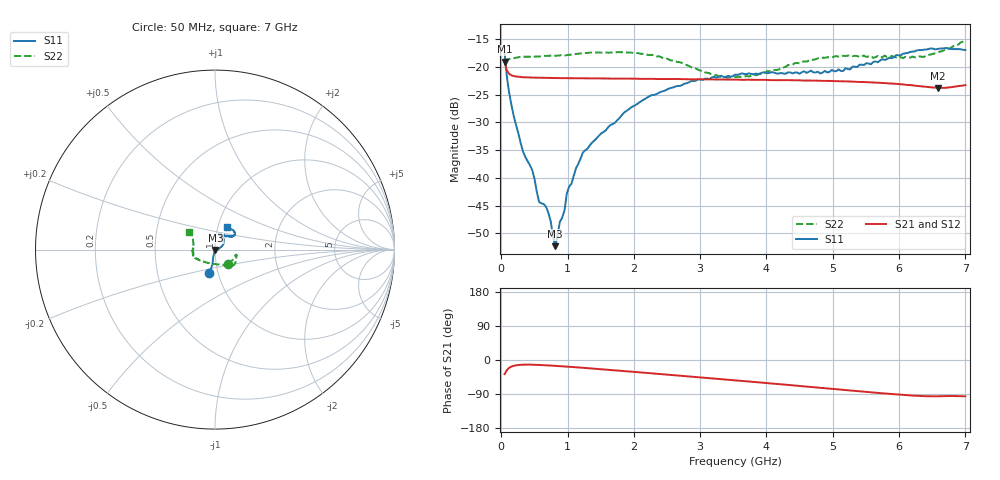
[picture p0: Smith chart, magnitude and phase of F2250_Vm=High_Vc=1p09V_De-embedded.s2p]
! Integrated Device Technology
! Corporate Headquarters
! 6024 Silver Creek Valley Road
! San Jose, CA 95138  USA
! Phone:  1-408-284-8200
! Toll Free:  1-800-223-1366
! Webpage:  http://www.idt.com/
! Timing and RF Division
! 515 Groton Road, Suite 102
! Westford, MA 01886-6024
! Device:  F2250
! Description: Voltage Variable RF Attenuator
! Frequency:  50.0 -  6000.00 MHz
! Package:  3x3 mm Thin QFN Plastic Package: 16 pin
! Ports:  2 RF, 3 DC
!  Pin  1  = GND
!  Pin  2  = NC
!  Pin  3  = RF1  = Port 1
!  Pin  4  = NC
!  Pin  5  = GND
!  Pin  6  = GND
!  Pin  7  = GND
!  Pin  8  = GND
!  Pin  9  = NC
!  Pin 10  = RF2  = Port 2
!  Pin 11  = NC
!  Pin 12  = GND
!  Pin 13  = GND
!  Pin 14  = VCNTRL
!  Pin 15  = VDD
!  Pin 16  = VMODE
! Vcntrl:  1.090 Volts
! Vmode:  +3.300 Volts
! Vdd:  +3.30  Volts
! Current:  1.330 mA
! Data:  The device was measured on a the F2250 evaluation board which has
!  individual transmission lines to the RF pins.  Data was collected
!  using a calibrated network analyzer.  The evaluation board was
!  de-embedded using a TRL calibration technique.
!  The reference plane is the edge of the package pin.
! Misc:  SN 10
!  Action Tracker AT0258
! Date Measured:  2014-11-26
! Date:  2015-10-15  MJV
! Note:
!  Integrated Device Technology supplies this data as a sample of measured
!  data at the package pin for this product.  Your particular data for this
!  product may vary.
!  Data was taken at 25 degrees C.
!  Integrated Device Technology reserves the right to change this data at anytime.
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# GHz S dB R 50
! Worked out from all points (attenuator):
!   201 points, 50 MHz to 7 GHz, reference 50 ohm
!   highest |S21| = -19.02 dB at 50 MHz (marker M1); lowest = -23.8 dB at 6.583 GHz (marker M2)
!   lowest |S11| = -52.3 dB at 814.5 MHz (marker M3), VSWR 1.00, Z = 50.2 - j0.147 ohm
!   |S11| at or under -10 dB: start of sweep to end of sweep
!   |S22| runs from -21.9 to -15.2 dB; largest |S21 - S12| = 0.00028
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0.05  -17.44 -103.4  -19.02 -37.3  -19.02 -37.3  -19.14 -48.2
0.08475  -21.81 -99.6  -20.68 -26.3  -20.67 -26.3  -18.63 -25.3
0.1195  -24.70 -101.4  -21.23 -20.5  -21.23 -20.5  -18.56 -18.0
0.29325  -33.75 -100.0  -21.80 -12.7  -21.82 -12.7  -18.12 -13.7
0.467  -38.59 -106.3  -21.92 -12.4  -21.90 -12.4  -18.18 -14.6
0.57125  -44.35 -95.6  -21.93 -13.0  -21.95 -13.1  -18.10 -17.0
0.64075  -44.72 -91.2  -21.94 -13.6  -21.94 -13.6  -17.98 -18.1
0.71025  -46.29 -79.8  -21.97 -14.3  -21.96 -14.3  -17.96 -19.9
0.8145  -52.31 -37.2  -21.99 -15.4  -21.98 -15.4  -17.98 -22.4
0.884  -47.88 -22.0  -22.01 -16.2  -21.98 -16.2  -17.89 -24.5
0.9535  -45.84 -30.4  -22.00 -17.0  -22.00 -17.0  -17.93 -25.6
0.98825  -42.84 -22.0  -22.00 -17.4  -22.00 -17.5  -17.86 -26.2
1.2315  -35.42 4.9  -22.02 -20.6  -22.03 -20.6  -17.47 -30.7
1.857  -28.16 23.9  -22.08 -29.3  -22.09 -29.3  -17.33 -39.1
2.37825  -24.63 36.2  -22.16 -36.7  -22.16 -36.7  -18.05 -46.5
2.86475  -22.51 49.6  -22.20 -43.9  -22.20 -43.9  -20.03 -59.4
3.525  -21.38 66.8  -22.27 -53.7  -22.26 -53.8  -21.81 -99.7
4.7065  -20.96 69.5  -22.45 -71.7  -22.43 -71.7  -18.68 -154.4
5.15825  -20.69 53.3  -22.58 -78.7  -22.57 -78.8  -17.96 -163.0
5.85325  -18.34 38.0  -22.96 -89.3  -22.95 -89.5  -18.25 -177.4
6.583  -16.73 43.1  -23.76 -95.7  -23.76 -95.8  -17.34 154.9
7  -16.93 61.9  -23.26 -95.8  -23.26 -95.9  -15.20 146.0
